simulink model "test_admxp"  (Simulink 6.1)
settings: Solver=ode45  StartTime=0.0  StopTime=2000  RelTol=1e-3
undefined symbols (not defined in the file or in its folder): Bit, Location, Lower, netlist, Width
libraries: xbsIndex_r3 x144, adlibrary2 x7

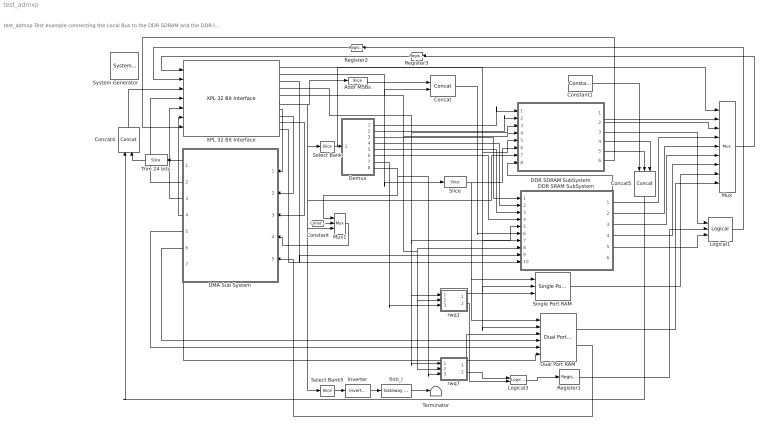
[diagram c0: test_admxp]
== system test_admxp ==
  note: test_admxp Test example connecting the Local Bus to the DDR SDRAM and the DDR-II SSRAM on the ADM-XP
  " System Generator" : xbsIndex_r3/ System Generator  Tag=genX  xilinxfamily=Virtex2P  part=xc2vp70  speed=-5  package=ff1704  synthesis_tool=XST  directory=./netlist  testbench=off  simulink_period=1  sysclk_period=10  incr_netlist=off  trim_vbits=Everywhere in SubSystem  dbl_ovrd=According to Block Masks  core_generation=According to Block Masks  run_coregen=off  deprecated_control=off  eval_field=0
  Addr MSBs : xbsIndex_r3/Slice  mode=Lower Bit Location + Width  nbits=5  bit1=0  base1=MSB of Input  bit0=4  base0=LSB of Input  boolean_output=off  explicit_period=on  period=1  dbl_ovrd=off
  Concat : xbsIndex_r3/Concat  num_inputs=2  explicit_period=on  period=1  dbl_ovrd=off
  Concat4 : xbsIndex_r3/Concat  Orientation=up  num_inputs=2  explicit_period=on  period=1  dbl_ovrd=off
  Concat5 : xbsIndex_r3/Concat  Orientation=down  num_inputs=3  explicit_period=on  period=1  dbl_ovrd=off
  Constant : xbsIndex_r3/Constant  const=0  equ=P=C  arith_type=Unsigned  n_bits=32  bin_pt=0  opselect=C  inp2=PCIN>>17  opr=+  inp1=P  carry=CIN  iostate=0  explicit_period=off  period=1  dbl_ovrd=off
  Constant1 : xbsIndex_r3/Constant  const=0  equ=P=C  arith_type=Unsigned  n_bits=6  bin_pt=0  opselect=C  inp2=PCIN>>17  opr=+  inp1=P  carry=CIN  iostate=0  explicit_period=on  period=1  dbl_ovrd=off
  DDR SDRAM SubSystem : Subsystem
  DDR SRAM SubSystem : Subsystem
  DMA Sub System : Subsystem  Orientation=left
  Demux : Subsystem
  Dual Port RAM : xbsIndex_r3/Dual Port RAM  depth=1024  initVector=sin(pi*(0:15)/16)  write_mode_A=Read After Write  write_mode_B=Read After Write  latency=1  mem_collision=off  init_zero=on  explicit_period=on  period=1  dbl_ovrd=off  rst_a=off  init_a=0  rst_b=off  init_b=0  show_param=off  distributed_mem=off  use_rpm=off  gen_core=off
  Inverter : xbsIndex_r3/Inverter  latency=0  explicit_period=off  period=1  en=off  dbl_ovrd=off  show_param=off
  Logical1 : xbsIndex_r3/Logical  logical_function=OR  inputs=3  precision=Full  arith_type=Unsigned  n_bits=8  bin_pt=2  align_bp=on  latency=0  explicit_period=off  period=1  en=off  dbl_ovrd=off  show_param=off
  Logical3 : xbsIndex_r3/Logical  logical_function=OR  inputs=2  precision=Full  arith_type=Unsigned  n_bits=8  bin_pt=2  align_bp=on  latency=0  explicit_period=off  period=1  en=off  dbl_ovrd=off  show_param=off
  Mux : xbsIndex_r3/Mux  inputs=8  precision=Full  arith_type="Signed  (2's comp)"  n_bits=8  bin_pt=2  quantization=Truncate  overflow=Wrap  latency=0  explicit_period=off  period=1  en=off  dbl_ovrd=off  show_param=off  mux_type=off  use_rpm=off  gen_core=off
  Mux1 : xbsIndex_r3/Mux  inputs=2  precision=Full  arith_type="Signed  (2's comp)"  n_bits=8  bin_pt=2  quantization=Truncate  overflow=Wrap  latency=0  explicit_period=off  period=1  en=off  dbl_ovrd=off  show_param=off  mux_type=off  use_rpm=off  gen_core=off
  Register1 : xbsIndex_r3/Register  init=0  reg_only_valid=off  explicit_period=off  period=1  rst=off  en=off  out_en=off  dbl_ovrd=off  show_param=off
  Register2 : xbsIndex_r3/Register  Orientation=left  init=0  reg_only_valid=off  explicit_period=on  period=1  rst=off  en=off  out_en=off  dbl_ovrd=off  show_param=off
  Register3 : xbsIndex_r3/Register  Orientation=left  init=0  reg_only_valid=off  explicit_period=on  period=1  rst=off  en=off  out_en=off  dbl_ovrd=off  show_param=off
  Select Bank : xbsIndex_r3/Slice  mode=Lower Bit Location + Width  nbits=3  bit1=0  base1=MSB of Input  bit0=0  base0=LSB of Input  boolean_output=off  explicit_period=on  period=1  dbl_ovrd=off
  Select Bank5 : xbsIndex_r3/Slice  mode=Lower Bit Location + Width  nbits=1  bit1=0  base1=MSB of Input  bit0=15  base0=LSB of Input  boolean_output=on  explicit_period=on  period=1  dbl_ovrd=off
  Single Port RAM : xbsIndex_r3/Single Port RAM  depth=1024  initVector=sin(pi*(0:15)/16)  write_mode=Read After Write  latency=1  init_zero=on  explicit_period=off  period=1  rst=off  init_reg=0  en=off  dbl_ovrd=off  show_param=off  distributed_mem=off  use_rpm=off  gen_core=off
  Slice : xbsIndex_r3/Slice  mode=Lower Bit Location + Width  nbits=10  bit1=0  base1=MSB of Input  bit0=0  base0=LSB of Input  boolean_output=off  explicit_period=on  period=1  dbl_ovrd=off
  Terminator : Terminator
  Trim 24 bits : xbsIndex_r3/Slice  Orientation=left  mode=Lower Bit Location + Width  nbits=24  bit1=0  base1=MSB of Input  bit0=0  base0=LSB of Input  boolean_output=off  explicit_period=on  period=1  dbl_ovrd=off
  XPL 32 Bit Interface : adlibrary2/ADM-XP/XPL 32 Bit Interface  program='load test_admxp_program.txt'  clock_ratio=1.5
  finti_l : xbsIndex_r3/Gateway Out  output_type=Double  nbits=8  bin_pt=6  arith_type=Boolean  quantization=Truncate  overflow=Wrap  hdl_port=on  timing_constraint=None  locs_specified=on  LOCs={'AF3'}  needs_fixed_name=off  show_param=off
  rwq1 : Subsystem
  rwq7 : Subsystem
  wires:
  XPL 32 Bit Interface/1 -> DDR SDRAM SubSystem/5(Data), DDR SRAM SubSystem/5(Data), Dual Port RAM/2, Single Port RAM/2
  Register1/1 -> Logical1/2
  Mux/1 -> Register3/1
  Register2/1 -> XPL 32 Bit Interface/2
  Register3/1 -> XPL 32 Bit Interface/1
  Slice/1 -> DDR SDRAM SubSystem/6(Cache Addr), Dual Port RAM/1, Single Port RAM/1
  Addr MSBs/1 -> Concat/1
  XPL 32 Bit Interface/2 -> Concat/2, Slice/1
  Select Bank/1 -> Demux/1(Select), Mux/1
  rwq7/1(wq) -> Dual Port RAM/3
  DMA Sub System/2(Read IFIFO) -> XPL 32 Bit Interface/4
  DMA Sub System/3(Write OFIFO) -> XPL 32 Bit Interface/5
  DMA Sub System/4(OFIFO_Data) -> XPL 32 Bit Interface/6
  Dual Port RAM/2 -> DMA Sub System/5(DP_RAM_Data)
  DMA Sub System/7(DP_RAM_WE) -> Dual Port RAM/6
  DMA Sub System/6(DP_RAM_Addr) -> Dual Port RAM/4
  DMA Sub System/5(DP_RAM_WData) -> Dual Port RAM/5
  Logical1/1 -> Register2/1
  XPL 32 Bit Interface/4 -> DDR SDRAM SubSystem/3(Write), DDR SRAM SubSystem/7(Write), rwq7/1(w), rwq1/1(w)
  XPL 32 Bit Interface/9 -> DMA Sub System/3(OFIFO_Full)
  XPL 32 Bit Interface/8 -> DMA Sub System/2(IFIFO_Empty)
  XPL 32 Bit Interface/7 -> DMA Sub System/1(IFIFO_Data)
  XPL 32 Bit Interface/6 -> Addr MSBs/1, Select Bank/1, DDR SDRAM SubSystem/7(Control), Select Bank5/1, Mux1/3
  XPL 32 Bit Interface/5 -> DDR SRAM SubSystem/8(Read), rwq7/2(r), rwq1/2(r), DDR SDRAM SubSystem/4(Read)
  Concat4/1 -> XPL 32 Bit Interface/3
  DMA Sub System/1(Status) -> Trim 24 bits/1
  Concat5/1 -> Concat4/1
  Select Bank5/1 -> Inverter/1
  finti_l/1 -> Terminator/1
  Concat/1 -> DDR SRAM SubSystem/6(Addr)
  Demux/1(En0) -> DDR SDRAM SubSystem/1(En0)
  Demux/3(En2) -> DDR SRAM SubSystem/1(En2)
  Demux/4(En3) -> DDR SRAM SubSystem/2(En3)
  Demux/5(En4) -> DDR SRAM SubSystem/3(En4)
  Demux/6(En5) -> DDR SRAM SubSystem/4(En5)
  DDR SRAM SubSystem/5(Data Valid) -> Logical1/3
  DDR SDRAM SubSystem/3(Data Valid) -> Logical1/1
  DDR SDRAM SubSystem/1(Data Out0) -> Mux/2
  DDR SDRAM SubSystem/2(Data Out1) -> Mux/3
  Dual Port RAM/1 -> Mux/9
  Demux/7(En6) -> rwq1/3(e)
  Demux/8(En7) -> rwq7/3(e), Mux1/1
  Demux/2(En1) -> DDR SDRAM SubSystem/2(En1)
  Mux1/1 -> DMA Sub System/4(Control)
  Constant/1 -> Mux1/2
  Trim 24 bits/1 -> Concat4/2
  DDR SRAM SubSystem/1(Data Out0) -> Mux/4
  DDR SRAM SubSystem/2(Data Out1) -> Mux/5
  DDR SRAM SubSystem/3(Data Out2) -> Mux/6
  DDR SRAM SubSystem/4(Data Out3) -> Mux/7
  XPL 32 Bit Interface/3 -> DDR SRAM SubSystem/9(be)
  rwq7/2(rq) -> Logical3/1
  Logical3/1 -> Register1/1
  rwq1/2(rq) -> Logical3/2
  rwq1/1(wq) -> Single Port RAM/3
  Single Port RAM/1 -> Mux/8
  XPL 32 Bit Interface/10 -> DDR SRAM SubSystem/10(ADLOCB_IN)
  DDR SRAM SubSystem/6(ADLOCB_OUT) -> DDR SDRAM SubSystem/8(ADLOCB_IN)
  DDR SDRAM SubSystem/6(ADLOCB_OUT) -> XPL 32 Bit Interface/7
  DDR SDRAM SubSystem/4(DDR_Busy0) -> Concat5/3
  DDR SDRAM SubSystem/5(DDR_Busy1) -> Concat5/2
  Constant1/1 -> Concat5/1
  Inverter/1 -> finti_l/1

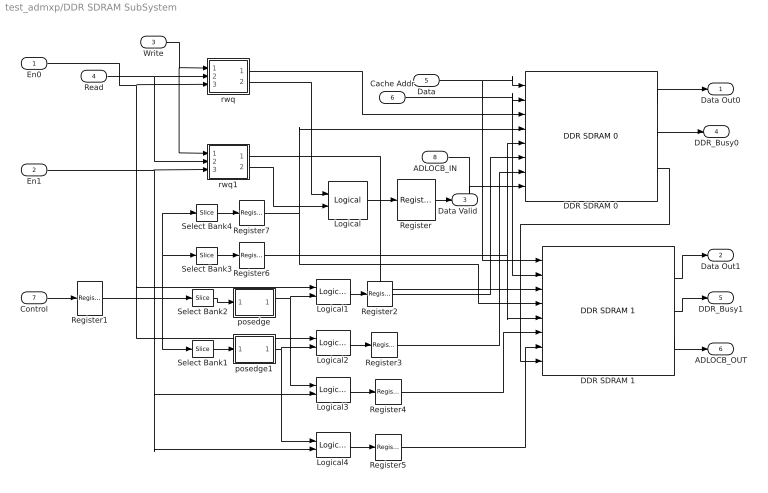
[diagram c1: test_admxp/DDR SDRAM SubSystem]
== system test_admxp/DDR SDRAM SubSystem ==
  En0 : Inport  Port=1  LatchInput=off
  En1 : Inport  Port=2  LatchInput=off
  Write : Inport  Port=3  LatchInput=off
  Read : Inport  Port=4  LatchInput=off
  Data : Inport  Port=5  LatchInput=off
  Cache Addr : Inport  Port=6  LatchInput=off
  Control : Inport  Port=7  LatchInput=off
  ADLOCB_IN : Inport  Port=8  LatchInput=off
  DDR SDRAM 0 : adlibrary2/ADM-XP/DDR SDRAM 0  memsize=1
  DDR SDRAM 1 : adlibrary2/ADM-XP/DDR SDRAM 1  memsize=1
  Logical : xbsIndex_r3/Logical  logical_function=OR  inputs=2  precision=Full  arith_type=Unsigned  n_bits=8  bin_pt=2  align_bp=on  latency=0  explicit_period=off  period=1  en=off  dbl_ovrd=off  show_param=off
  Logical{1..4} (4 alike) : xbsIndex_r3/Logical  logical_function=AND  inputs=2  precision=Full  arith_type=Unsigned  n_bits=8  bin_pt=2  align_bp=on  latency=0  explicit_period=off  period=1  en=off  dbl_ovrd=off  show_param=off
  Register{,2..7} (7 alike) : xbsIndex_r3/Register  init=0  reg_only_valid=off  explicit_period=on  period=1  rst=off  en=off  out_en=off  dbl_ovrd=off  show_param=off
  Register1 : xbsIndex_r3/Register  init=0  reg_only_valid=off  explicit_period=off  period=1  rst=off  en=off  out_en=off  dbl_ovrd=off  show_param=off
  Select Bank1 : xbsIndex_r3/Slice  mode=Lower Bit Location + Width  nbits=1  bit1=0  base1=MSB of Input  bit0=5  base0=LSB of Input  boolean_output=on  explicit_period=on  period=1  dbl_ovrd=off
  Select Bank2 : xbsIndex_r3/Slice  mode=Lower Bit Location + Width  nbits=1  bit1=0  base1=MSB of Input  bit0=4  base0=LSB of Input  boolean_output=on  explicit_period=on  period=1  dbl_ovrd=off
  Select Bank3 : xbsIndex_r3/Slice  mode=Lower Bit Location + Width  nbits=4  bit1=0  base1=MSB of Input  bit0=8  base0=LSB of Input  boolean_output=off  explicit_period=on  period=1  dbl_ovrd=off
  Select Bank4 : xbsIndex_r3/Slice  mode=Lower Bit Location + Width  nbits=15  bit1=0  base1=MSB of Input  bit0=16  base0=LSB of Input  boolean_output=off  explicit_period=on  period=1  dbl_ovrd=off
  posedge : Subsystem
  posedge1 : Subsystem
  rwq : Subsystem
  rwq1 : Subsystem
  Data Out0 : Outport
  Data Out1 : Outport  Port=2
  Data Valid : Outport  Port=3
  DDR_Busy0 : Outport  Port=4
  DDR_Busy1 : Outport  Port=5
  ADLOCB_OUT : Outport  Port=6
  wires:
  DDR SDRAM 0/1 -> Data Out0/1
  DDR SDRAM 0/2 -> DDR_Busy0/1
  En0/1 -> rwq/3(e), Logical1/1, Logical2/1
  En1/1 -> rwq1/3(e), Logical4/2, Logical3/2
  Write/1 -> rwq/1(w), rwq1/1(w)
  Read/1 -> rwq/2(r), rwq1/2(r)
  Data/1 -> DDR SDRAM 0/1, DDR SDRAM 1/1
  Cache Addr/1 -> DDR SDRAM 0/2, DDR SDRAM 1/2
  rwq/1(wq) -> DDR SDRAM 0/3
  rwq1/1(wq) -> DDR SDRAM 1/3
  Logical/1 -> Register/1
  Register/1 -> Data Valid/1
  rwq/2(rq) -> Logical/1
  rwq1/2(rq) -> Logical/2
  Control/1 -> Register1/1
  Select Bank2/1 -> posedge/1(In1)
  Select Bank1/1 -> posedge1/1(In1)
  posedge/1(Out1) -> Logical1/2, Logical3/1
  posedge1/1(Out1) -> Logical2/2, Logical4/1
  Logical1/1 -> Register2/1
  Logical2/1 -> Register3/1
  Logical3/1 -> Register4/1
  Register1/1 -> Select Bank2/1, Select Bank1/1, Select Bank4/1, Select Bank3/1
  Select Bank3/1 -> Register6/1
  Select Bank4/1 -> Register7/1
  Logical4/1 -> Register5/1
  DDR SDRAM 1/1 -> Data Out1/1
  DDR SDRAM 1/2 -> DDR_Busy1/1
  Register2/1 -> DDR SDRAM 0/6
  Register3/1 -> DDR SDRAM 0/7
  Register4/1 -> DDR SDRAM 1/6
  Register5/1 -> DDR SDRAM 1/7
  Register6/1 -> DDR SDRAM 0/5, DDR SDRAM 1/5
  Register7/1 -> DDR SDRAM 0/4, DDR SDRAM 1/4
  ADLOCB_IN/1 -> DDR SDRAM 0/8
  DDR SDRAM 0/3 -> DDR SDRAM 1/8
  DDR SDRAM 1/3 -> ADLOCB_OUT/1

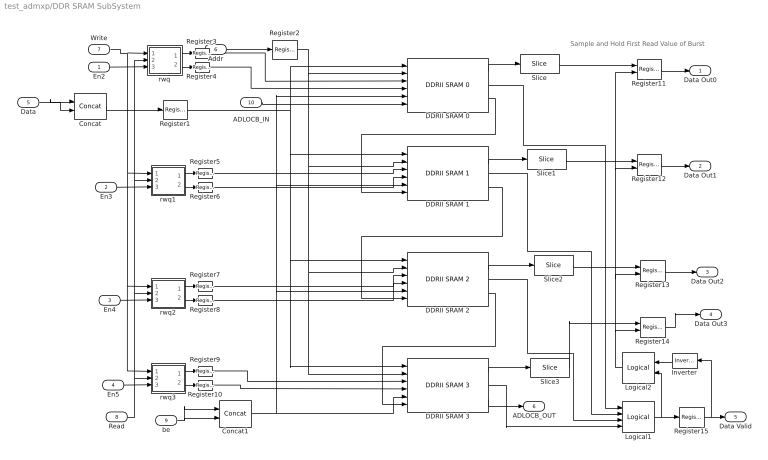
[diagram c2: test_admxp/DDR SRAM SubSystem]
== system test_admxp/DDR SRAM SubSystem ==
  note: Sample and Hold First Read Value of Burst
  En2 : Inport  Port=1  LatchInput=off
  En3 : Inport  Port=2  LatchInput=off
  En4 : Inport  Port=3  LatchInput=off
  En5 : Inport  Port=4  LatchInput=off
  Data : Inport  Port=5  LatchInput=off
  Addr : Inport  Port=6  LatchInput=off
  Write : Inport  Port=7  LatchInput=off
  Read : Inport  Port=8  LatchInput=off
  be : Inport  Port=9  LatchInput=off
  ADLOCB_IN : Inport  Port=10  LatchInput=off
  Concat : xbsIndex_r3/Concat  num_inputs=2  explicit_period=on  period=1  dbl_ovrd=off
  Concat1 : xbsIndex_r3/Concat  num_inputs=2  explicit_period=on  period=1  dbl_ovrd=off
  DDRII SRAM 0 : adlibrary2/ADM-XP/DDRII SRAM 0
  DDRII SRAM 1 : adlibrary2/ADM-XP/DDRII SRAM 1
  DDRII SRAM 2 : adlibrary2/ADM-XP/DDRII SRAM 2
  DDRII SRAM 3 : adlibrary2/ADM-XP/DDRII SRAM 3
  Inverter : xbsIndex_r3/Inverter  Orientation=left  latency=0  explicit_period=off  period=1  en=off  dbl_ovrd=off  show_param=off
  Logical1 : xbsIndex_r3/Logical  logical_function=OR  inputs=4  precision=Full  arith_type=Unsigned  n_bits=8  bin_pt=2  align_bp=on  latency=0  explicit_period=off  period=1  en=off  dbl_ovrd=off  show_param=off
  Logical2 : xbsIndex_r3/Logical  Orientation=left  logical_function=AND  inputs=2  precision=Full  arith_type=Unsigned  n_bits=8  bin_pt=2  align_bp=on  latency=0  explicit_period=off  period=1  en=off  dbl_ovrd=off  show_param=off
  Register{1..10,15} (11 alike) : xbsIndex_r3/Register  init=0  reg_only_valid=off  explicit_period=off  period=1  rst=off  en=off  out_en=off  dbl_ovrd=off  show_param=off
  Register{11..14} (4 alike) : xbsIndex_r3/Register  init=0  reg_only_valid=off  explicit_period=off  period=1  rst=off  en=on  out_en=off  dbl_ovrd=off  show_param=off
  Slice{,1..3} (4 alike) : xbsIndex_r3/Slice  mode=Lower Bit Location + Width  nbits=32  bit1=0  base1=MSB of Input  bit0=0  base0=LSB of Input  boolean_output=off  explicit_period=on  period=1  dbl_ovrd=off
  rwq : Subsystem
  rwq1 : Subsystem
  rwq2 : Subsystem
  rwq3 : Subsystem
  Data Out0 : Outport
  Data Out1 : Outport  Port=2
  Data Out2 : Outport  Port=3
  Data Out3 : Outport  Port=4
  Data Valid : Outport  Port=5
  ADLOCB_OUT : Outport  Port=6
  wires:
  En5/1 -> rwq3/3(e)
  En4/1 -> rwq2/3(e)
  En3/1 -> rwq1/3(e)
  En2/1 -> rwq/3(e)
  Write/1 -> rwq/1(w), rwq3/1(w), rwq2/1(w), rwq1/1(w)
  Read/1 -> rwq3/2(r), rwq/2(r), rwq1/2(r), rwq2/2(r)
  Concat/1 -> Register1/1
  Data/1 -> Concat/1, Concat/2
  Addr/1 -> Register2/1
  rwq/1(wq) -> Register3/1
  rwq/2(rq) -> Register4/1
  rwq1/1(wq) -> Register5/1
  rwq1/2(rq) -> Register6/1
  rwq2/1(wq) -> Register7/1
  rwq2/2(rq) -> Register8/1
  rwq3/1(wq) -> Register9/1
  rwq3/2(rq) -> Register10/1
  be/1 -> Concat1/1, Concat1/2
  DDRII SRAM 0/1 -> Slice/1
  DDRII SRAM 1/1 -> Slice1/1
  DDRII SRAM 2/1 -> Slice2/1
  DDRII SRAM 3/1 -> Slice3/1
  DDRII SRAM 3/2 -> Logical1/4
  Logical1/1 -> Register15/1, Logical2/2
  DDRII SRAM 2/2 -> Logical1/3
  DDRII SRAM 1/2 -> Logical1/2
  DDRII SRAM 0/2 -> Logical1/1
  ADLOCB_IN/1 -> DDRII SRAM 0/6
  DDRII SRAM 0/3 -> DDRII SRAM 1/6
  DDRII SRAM 1/3 -> DDRII SRAM 2/6
  DDRII SRAM 2/3 -> DDRII SRAM 3/6
  DDRII SRAM 3/3 -> ADLOCB_OUT/1
  Concat1/1 -> DDRII SRAM 3/5, DDRII SRAM 2/5, DDRII SRAM 1/5, DDRII SRAM 0/5
  Register1/1 -> DDRII SRAM 0/1, DDRII SRAM 1/1, DDRII SRAM 2/1, DDRII SRAM 3/1
  Register2/1 -> DDRII SRAM 0/2, DDRII SRAM 1/2, DDRII SRAM 2/2, DDRII SRAM 3/2
  Register3/1 -> DDRII SRAM 0/3
  Register4/1 -> DDRII SRAM 0/4
  Register5/1 -> DDRII SRAM 1/3
  Register6/1 -> DDRII SRAM 1/4
  Register7/1 -> DDRII SRAM 2/3
  Register8/1 -> DDRII SRAM 2/4
  Register9/1 -> DDRII SRAM 3/3
  Register10/1 -> DDRII SRAM 3/4
  Slice/1 -> Register11/1
  Register11/1 -> Data Out0/1
  Register12/1 -> Data Out1/1
  Slice1/1 -> Register12/1
  Slice2/1 -> Register13/1
  Register13/1 -> Data Out2/1
  Slice3/1 -> Register14/1
  Register14/1 -> Data Out3/1
  Register15/1 -> Data Valid/1, Inverter/1
  Logical2/1 -> Register14/2, Register13/2, Register12/2, Register11/2
  Inverter/1 -> Logical2/1

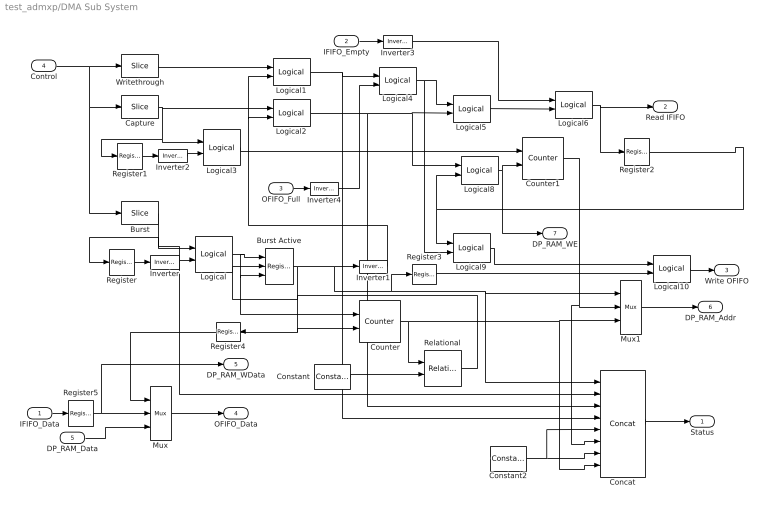
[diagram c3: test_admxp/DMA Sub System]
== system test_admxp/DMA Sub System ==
  IFIFO_Data : Inport  Port=1  LatchInput=off
  IFIFO_Empty : Inport  Port=2  LatchInput=off
  OFIFO_Full : Inport  Port=3  LatchInput=off
  Control : Inport  Port=4  LatchInput=off
  DP_RAM_Data : Inport  Port=5  LatchInput=off
  Burst : xbsIndex_r3/Slice  mode=Lower Bit Location + Width  nbits=1  bit1=0  base1=MSB of Input  bit0=6  base0=LSB of Input  boolean_output=on  explicit_period=on  period=1  dbl_ovrd=off
  Burst Active : xbsIndex_r3/Register  init=0  reg_only_valid=off  explicit_period=on  period=1  rst=on  en=on  out_en=off  dbl_ovrd=off  show_param=off
  Capture : xbsIndex_r3/Slice  mode=Lower Bit Location + Width  nbits=1  bit1=0  base1=MSB of Input  bit0=5  base0=LSB of Input  boolean_output=on  explicit_period=on  period=1  dbl_ovrd=off
  Concat : xbsIndex_r3/Concat  num_inputs=8  explicit_period=on  period=1  dbl_ovrd=off
  Constant : xbsIndex_r3/Constant  const=511  equ=P=C  arith_type=Unsigned  n_bits=10  bin_pt=0  opselect=C  inp2=PCIN>>17  opr=+  inp1=P  carry=CIN  iostate=0  explicit_period=off  period=1  dbl_ovrd=off
  Constant2 : xbsIndex_r3/Constant  const=0  equ=P=C  arith_type=Unsigned  n_bits=2  bin_pt=0  opselect=C  inp2=PCIN>>17  opr=+  inp1=P  carry=CIN  iostate=0  explicit_period=off  period=1  dbl_ovrd=off
  Counter : xbsIndex_r3/Counter  cnt_type=Count Limited  n_bits=10  bin_pt=0  arith_type=Unsigned  start_count=0  cnt_to=Inf  cnt_by_val=1  operation=Up  explicit_period=on  period=1  load_pin=off  rst=on  en=on  dbl_ovrd=off  show_param=off  use_rpm=on  gen_core=off
  Counter1 : xbsIndex_r3/Counter  cnt_type=Count Limited  n_bits=10  bin_pt=0  arith_type=Unsigned  start_count=0  cnt_to=Inf  cnt_by_val=1  operation=Up  explicit_period=on  period=1  load_pin=off  rst=on  en=on  dbl_ovrd=off  show_param=off  use_rpm=on  gen_core=off
  Inverter{,1..2,4} (4 alike) : xbsIndex_r3/Inverter  latency=0  explicit_period=off  period=1  en=off  dbl_ovrd=off  show_param=off
  Inverter3 : xbsIndex_r3/Inverter  latency=0  explicit_period=on  period=1  en=off  dbl_ovrd=off  show_param=off
  Logical : xbsIndex_r3/Logical  logical_function=AND  inputs=2  precision=Full  arith_type=Unsigned  n_bits=8  bin_pt=2  align_bp=on  latency=0  explicit_period=on  period=1  en=off  dbl_ovrd=off  show_param=off
  Logical{1..2,4,8..9} (5 alike) : xbsIndex_r3/Logical  logical_function=AND  inputs=2  precision=Full  arith_type=Unsigned  n_bits=8  bin_pt=2  align_bp=on  latency=0  explicit_period=off  period=1  en=off  dbl_ovrd=off  show_param=off
  Logical10 : xbsIndex_r3/Logical  logical_function=OR  inputs=2  precision=Full  arith_type=Unsigned  n_bits=8  bin_pt=2  align_bp=on  latency=0  explicit_period=on  period=1  en=off  dbl_ovrd=off  show_param=off
  Logical3 : xbsIndex_r3/Logical  logical_function=AND  inputs=2  precision=Full  arith_type=Unsigned  n_bits=8  bin_pt=2  align_bp=on  latency=0  explicit_period=on  period=1  en=off  dbl_ovrd=off  show_param=off
  Logical5 : xbsIndex_r3/Logical  logical_function=OR  inputs=2  precision=Full  arith_type=Unsigned  n_bits=8  bin_pt=2  align_bp=on  latency=0  explicit_period=off  period=1  en=off  dbl_ovrd=off  show_param=off
  Logical6 : xbsIndex_r3/Logical  logical_function=AND  inputs=2  precision=Full  arith_type=Unsigned  n_bits=8  bin_pt=2  align_bp=on  latency=0  explicit_period=on  period=1  en=off  dbl_ovrd=off  show_param=off
  Mux : xbsIndex_r3/Mux  inputs=2  precision=Full  arith_type="Signed  (2's comp)"  n_bits=8  bin_pt=2  quantization=Truncate  overflow=Wrap  latency=0  explicit_period=on  period=1  en=off  dbl_ovrd=off  show_param=off  mux_type=off  use_rpm=off  gen_core=off
  Mux1 : xbsIndex_r3/Mux  inputs=2  precision=Full  arith_type="Signed  (2's comp)"  n_bits=8  bin_pt=2  quantization=Truncate  overflow=Wrap  latency=0  explicit_period=off  period=1  en=off  dbl_ovrd=off  show_param=off  mux_type=off  use_rpm=off  gen_core=off
  Register{,1..3,5} (5 alike) : xbsIndex_r3/Register  init=0  reg_only_valid=off  explicit_period=on  period=1  rst=off  en=off  out_en=off  dbl_ovrd=off  show_param=off
  Register4 : xbsIndex_r3/Register  Orientation=left  init=0  reg_only_valid=off  explicit_period=on  period=1  rst=off  en=off  out_en=off  dbl_ovrd=off  show_param=off
  Relational : xbsIndex_r3/Relational  mode=a=b  latency=0  explicit_period=off  period=1  en=off  dbl_ovrd=off  show_param=off
  Writethrough : xbsIndex_r3/Slice  mode=Lower Bit Location + Width  nbits=1  bit1=0  base1=MSB of Input  bit0=4  base0=LSB of Input  boolean_output=on  explicit_period=on  period=1  dbl_ovrd=off
  Status : Outport
  Read IFIFO : Outport  Port=2
  Write OFIFO : Outport  Port=3
  OFIFO_Data : Outport  Port=4
  DP_RAM_WData : Outport  Port=5
  DP_RAM_Addr : Outport  Port=6
  DP_RAM_WE : Outport  Port=7
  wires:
  Mux/1 -> OFIFO_Data/1
  IFIFO_Data/1 -> Register5/1
  DP_RAM_Data/1 -> Mux/3
  Control/1 -> Writethrough/1, Burst/1, Capture/1
  Burst/1 -> Register/1, Logical/1, Concat/2
  Register/1 -> Inverter/1
  Inverter/1 -> Logical/2
  Logical/1 -> Burst Active/1, Burst Active/3, Counter/1
  Burst Active/1 -> Inverter1/1, Register3/1, Mux1/1, Concat/1, Counter/2, Register4/1
  Inverter1/1 -> Logical1/2, Logical2/2
  Capture/1 -> Logical2/1, Logical3/1, Register1/1
  Writethrough/1 -> Logical1/1
  Register1/1 -> Inverter2/1
  Inverter2/1 -> Logical3/2
  Logical3/1 -> Counter1/1
  IFIFO_Empty/1 -> Inverter3/1
  OFIFO_Full/1 -> Inverter4/1
  Logical1/1 -> Logical4/1, Concat/4
  Inverter4/1 -> Logical4/2
  Logical2/1 -> Logical5/2, Logical8/1, Concat/3
  Logical4/1 -> Logical5/1, Logical9/2
  Inverter3/1 -> Logical6/1
  Logical5/1 -> Logical6/2
  Logical6/1 -> Read IFIFO/1, Register2/1
  Register2/1 -> Logical8/2, Logical9/1
  Logical8/1 -> Counter1/2, DP_RAM_WE/1
  Mux1/1 -> DP_RAM_Addr/1
  Counter1/1 -> Mux1/2, Concat/6
  Counter/1 -> Relational/1, Mux1/3, Concat/8
  Logical9/1 -> Logical10/1
  Register3/1 -> Logical10/2
  Constant/1 -> Relational/2
  Relational/1 -> Burst Active/2
  Constant2/1 -> Concat/5, Concat/7
  Concat/1 -> Status/1
  Logical10/1 -> Write OFIFO/1
  Register4/1 -> Mux/1
  Register5/1 -> Mux/2, DP_RAM_WData/1

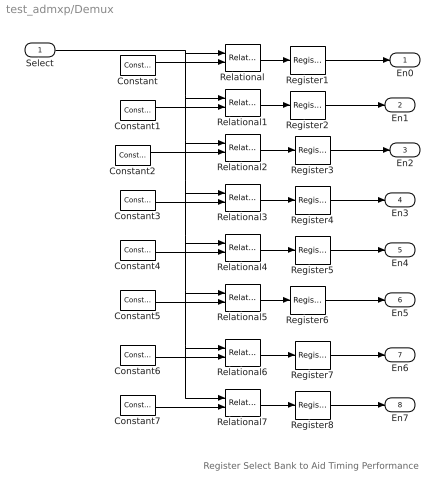
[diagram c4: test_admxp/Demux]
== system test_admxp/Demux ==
  note: Register Select Bank to Aid Timing Performance
  Select : Inport  Port=1  LatchInput=off
  Constant : xbsIndex_r3/Constant  const=0  equ=P=C  arith_type=Unsigned  n_bits=3  bin_pt=0  opselect=C  inp2=PCIN>>17  opr=+  inp1=P  carry=CIN  iostate=0  explicit_period=off  period=1  dbl_ovrd=off
  Constant1 : xbsIndex_r3/Constant  const=1  equ=P=C  arith_type=Unsigned  n_bits=3  bin_pt=0  opselect=C  inp2=PCIN>>17  opr=+  inp1=P  carry=CIN  iostate=0  explicit_period=off  period=1  dbl_ovrd=off
  Constant2 : xbsIndex_r3/Constant  const=2  equ=P=C  arith_type=Unsigned  n_bits=3  bin_pt=0  opselect=C  inp2=PCIN>>17  opr=+  inp1=P  carry=CIN  iostate=0  explicit_period=off  period=1  dbl_ovrd=off
  Constant3 : xbsIndex_r3/Constant  const=3  equ=P=C  arith_type=Unsigned  n_bits=3  bin_pt=0  opselect=C  inp2=PCIN>>17  opr=+  inp1=P  carry=CIN  iostate=0  explicit_period=off  period=1  dbl_ovrd=off
  Constant4 : xbsIndex_r3/Constant  const=4  equ=P=C  arith_type=Unsigned  n_bits=3  bin_pt=0  opselect=C  inp2=PCIN>>17  opr=+  inp1=P  carry=CIN  iostate=0  explicit_period=off  period=1  dbl_ovrd=off
  Constant5 : xbsIndex_r3/Constant  const=5  equ=P=C  arith_type=Unsigned  n_bits=3  bin_pt=0  opselect=C  inp2=PCIN>>17  opr=+  inp1=P  carry=CIN  iostate=0  explicit_period=off  period=1  dbl_ovrd=off
  Constant6 : xbsIndex_r3/Constant  const=6  equ=P=C  arith_type=Unsigned  n_bits=3  bin_pt=0  opselect=C  inp2=PCIN>>17  opr=+  inp1=P  carry=CIN  iostate=0  explicit_period=off  period=1  dbl_ovrd=off
  Constant7 : xbsIndex_r3/Constant  const=7  equ=P=C  arith_type=Unsigned  n_bits=3  bin_pt=0  opselect=C  inp2=PCIN>>17  opr=+  inp1=P  carry=CIN  iostate=0  explicit_period=off  period=1  dbl_ovrd=off
  Register{1..8} (8 alike) : xbsIndex_r3/Register  init=0  reg_only_valid=off  explicit_period=off  period=1  rst=off  en=off  out_en=off  dbl_ovrd=off  show_param=off
  Relational{,1..7} (8 alike) : xbsIndex_r3/Relational  mode=a=b  latency=0  explicit_period=off  period=1  en=off  dbl_ovrd=off  show_param=off
  En0 : Outport
  En1 : Outport  Port=2
  En2 : Outport  Port=3
  En3 : Outport  Port=4
  En4 : Outport  Port=5
  En5 : Outport  Port=6
  En6 : Outport  Port=7
  En7 : Outport  Port=8
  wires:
  Relational/1 -> Register1/1
  Relational1/1 -> Register2/1
  Relational2/1 -> Register3/1
  Relational3/1 -> Register4/1
  Select/1 -> Relational/1, Relational1/1, Relational2/1, Relational3/1, Relational4/1, Relational5/1, Relational6/1, Relational7/1
  Constant/1 -> Relational/2
  Constant1/1 -> Relational1/2
  Constant2/1 -> Relational2/2
  Constant3/1 -> Relational3/2
  Relational4/1 -> Register5/1
  Constant4/1 -> Relational4/2
  Relational5/1 -> Register6/1
  Constant5/1 -> Relational5/2
  Relational6/1 -> Register7/1
  Constant6/1 -> Relational6/2
  Relational7/1 -> Register8/1
  Constant7/1 -> Relational7/2
  Register1/1 -> En0/1
  Register2/1 -> En1/1
  Register3/1 -> En2/1
  Register4/1 -> En3/1
  Register5/1 -> En4/1
  Register6/1 -> En5/1
  Register7/1 -> En6/1
  Register8/1 -> En7/1

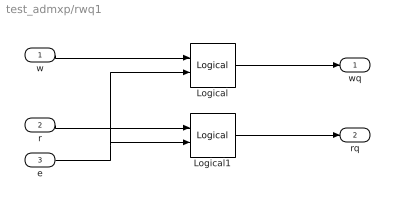
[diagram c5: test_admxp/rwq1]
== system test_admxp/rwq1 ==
  w : Inport  Port=1  LatchInput=off
  r : Inport  Port=2  LatchInput=off
  e : Inport  Port=3  LatchInput=off
  Logical : xbsIndex_r3/Logical  logical_function=AND  inputs=2  precision=Full  arith_type=Unsigned  n_bits=8  bin_pt=2  align_bp=on  latency=0  explicit_period=off  period=1  en=off  dbl_ovrd=off  show_param=off
  Logical1 : xbsIndex_r3/Logical  logical_function=AND  inputs=2  precision=Full  arith_type=Unsigned  n_bits=8  bin_pt=2  align_bp=on  latency=0  explicit_period=off  period=1  en=off  dbl_ovrd=off  show_param=off
  wq : Outport
  rq : Outport  Port=2
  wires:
  e/1 -> Logical1/2, Logical/2
  r/1 -> Logical1/1
  w/1 -> Logical/1
  Logical/1 -> wq/1
  Logical1/1 -> rq/1

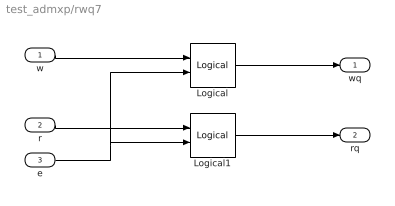
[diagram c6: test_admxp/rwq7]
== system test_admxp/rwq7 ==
  w : Inport  Port=1  LatchInput=off
  r : Inport  Port=2  LatchInput=off
  e : Inport  Port=3  LatchInput=off
  Logical : xbsIndex_r3/Logical  logical_function=AND  inputs=2  precision=Full  arith_type=Unsigned  n_bits=8  bin_pt=2  align_bp=on  latency=0  explicit_period=off  period=1  en=off  dbl_ovrd=off  show_param=off
  Logical1 : xbsIndex_r3/Logical  logical_function=AND  inputs=2  precision=Full  arith_type=Unsigned  n_bits=8  bin_pt=2  align_bp=on  latency=0  explicit_period=off  period=1  en=off  dbl_ovrd=off  show_param=off
  wq : Outport
  rq : Outport  Port=2
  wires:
  e/1 -> Logical1/2, Logical/2
  r/1 -> Logical1/1
  w/1 -> Logical/1
  Logical/1 -> wq/1
  Logical1/1 -> rq/1

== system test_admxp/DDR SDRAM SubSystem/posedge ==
  In1 : Inport  Port=1  LatchInput=off
  Inverter : xbsIndex_r3/Inverter  latency=0  explicit_period=off  period=1  en=off  dbl_ovrd=off  show_param=off
  Logical : xbsIndex_r3/Logical  logical_function=AND  inputs=2  precision=Full  arith_type=Unsigned  n_bits=8  bin_pt=2  align_bp=on  latency=0  explicit_period=off  period=1  en=off  dbl_ovrd=off  show_param=off
  Register : xbsIndex_r3/Register  init=0  reg_only_valid=off  explicit_period=on  period=1  rst=off  en=off  out_en=off  dbl_ovrd=off  show_param=off
  Register1 : xbsIndex_r3/Register  init=0  reg_only_valid=off  explicit_period=on  period=1  rst=off  en=off  out_en=off  dbl_ovrd=off  show_param=off
  Out1 : Outport
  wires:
  Inverter/1 -> Logical/1
  Logical/1 -> Out1/1
  Register/1 -> Logical/2
  In1/1 -> Register1/1
  Register1/1 -> Inverter/1, Register/1

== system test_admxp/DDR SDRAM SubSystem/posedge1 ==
  In1 : Inport  Port=1  LatchInput=off
  Inverter : xbsIndex_r3/Inverter  latency=0  explicit_period=off  period=1  en=off  dbl_ovrd=off  show_param=off
  Logical : xbsIndex_r3/Logical  logical_function=AND  inputs=2  precision=Full  arith_type=Unsigned  n_bits=8  bin_pt=2  align_bp=on  latency=0  explicit_period=off  period=1  en=off  dbl_ovrd=off  show_param=off
  Register : xbsIndex_r3/Register  init=0  reg_only_valid=off  explicit_period=on  period=1  rst=off  en=off  out_en=off  dbl_ovrd=off  show_param=off
  Register1 : xbsIndex_r3/Register  init=0  reg_only_valid=off  explicit_period=on  period=1  rst=off  en=off  out_en=off  dbl_ovrd=off  show_param=off
  Out1 : Outport
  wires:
  Inverter/1 -> Logical/1
  Logical/1 -> Out1/1
  Register/1 -> Logical/2
  In1/1 -> Register1/1
  Register1/1 -> Inverter/1, Register/1

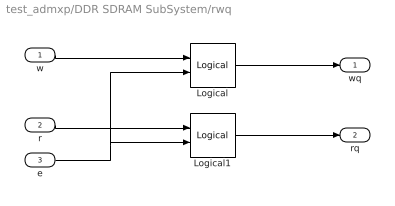
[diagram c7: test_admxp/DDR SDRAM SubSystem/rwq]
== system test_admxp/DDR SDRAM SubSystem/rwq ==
  w : Inport  Port=1  LatchInput=off
  r : Inport  Port=2  LatchInput=off
  e : Inport  Port=3  LatchInput=off
  Logical : xbsIndex_r3/Logical  logical_function=AND  inputs=2  precision=Full  arith_type=Unsigned  n_bits=8  bin_pt=2  align_bp=on  latency=0  explicit_period=off  period=1  en=off  dbl_ovrd=off  show_param=off
  Logical1 : xbsIndex_r3/Logical  logical_function=AND  inputs=2  precision=Full  arith_type=Unsigned  n_bits=8  bin_pt=2  align_bp=on  latency=0  explicit_period=off  period=1  en=off  dbl_ovrd=off  show_param=off
  wq : Outport
  rq : Outport  Port=2
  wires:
  e/1 -> Logical1/2, Logical/2
  r/1 -> Logical1/1
  w/1 -> Logical/1
  Logical/1 -> wq/1
  Logical1/1 -> rq/1

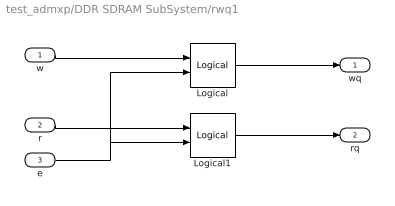
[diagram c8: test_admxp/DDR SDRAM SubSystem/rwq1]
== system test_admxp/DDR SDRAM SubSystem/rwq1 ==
  w : Inport  Port=1  LatchInput=off
  r : Inport  Port=2  LatchInput=off
  e : Inport  Port=3  LatchInput=off
  Logical : xbsIndex_r3/Logical  logical_function=AND  inputs=2  precision=Full  arith_type=Unsigned  n_bits=8  bin_pt=2  align_bp=on  latency=0  explicit_period=off  period=1  en=off  dbl_ovrd=off  show_param=off
  Logical1 : xbsIndex_r3/Logical  logical_function=AND  inputs=2  precision=Full  arith_type=Unsigned  n_bits=8  bin_pt=2  align_bp=on  latency=0  explicit_period=off  period=1  en=off  dbl_ovrd=off  show_param=off
  wq : Outport
  rq : Outport  Port=2
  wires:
  e/1 -> Logical1/2, Logical/2
  r/1 -> Logical1/1
  w/1 -> Logical/1
  Logical/1 -> wq/1
  Logical1/1 -> rq/1

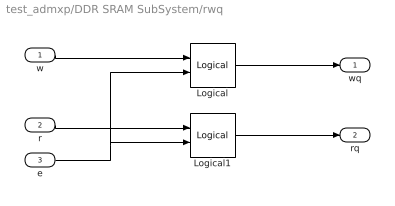
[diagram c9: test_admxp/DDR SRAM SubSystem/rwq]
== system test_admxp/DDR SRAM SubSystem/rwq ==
  w : Inport  Port=1  LatchInput=off
  r : Inport  Port=2  LatchInput=off
  e : Inport  Port=3  LatchInput=off
  Logical : xbsIndex_r3/Logical  logical_function=AND  inputs=2  precision=Full  arith_type=Unsigned  n_bits=8  bin_pt=2  align_bp=on  latency=0  explicit_period=off  period=1  en=off  dbl_ovrd=off  show_param=off
  Logical1 : xbsIndex_r3/Logical  logical_function=AND  inputs=2  precision=Full  arith_type=Unsigned  n_bits=8  bin_pt=2  align_bp=on  latency=0  explicit_period=off  period=1  en=off  dbl_ovrd=off  show_param=off
  wq : Outport
  rq : Outport  Port=2
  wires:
  e/1 -> Logical1/2, Logical/2
  r/1 -> Logical1/1
  w/1 -> Logical/1
  Logical/1 -> wq/1
  Logical1/1 -> rq/1

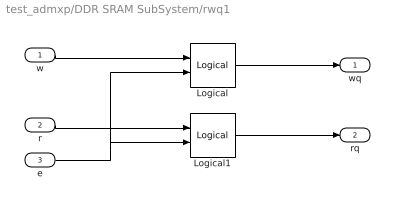
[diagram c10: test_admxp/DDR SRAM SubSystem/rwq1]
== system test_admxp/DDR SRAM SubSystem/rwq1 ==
  w : Inport  Port=1  LatchInput=off
  r : Inport  Port=2  LatchInput=off
  e : Inport  Port=3  LatchInput=off
  Logical : xbsIndex_r3/Logical  logical_function=AND  inputs=2  precision=Full  arith_type=Unsigned  n_bits=8  bin_pt=2  align_bp=on  latency=0  explicit_period=off  period=1  en=off  dbl_ovrd=off  show_param=off
  Logical1 : xbsIndex_r3/Logical  logical_function=AND  inputs=2  precision=Full  arith_type=Unsigned  n_bits=8  bin_pt=2  align_bp=on  latency=0  explicit_period=off  period=1  en=off  dbl_ovrd=off  show_param=off
  wq : Outport
  rq : Outport  Port=2
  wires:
  e/1 -> Logical1/2, Logical/2
  r/1 -> Logical1/1
  w/1 -> Logical/1
  Logical/1 -> wq/1
  Logical1/1 -> rq/1

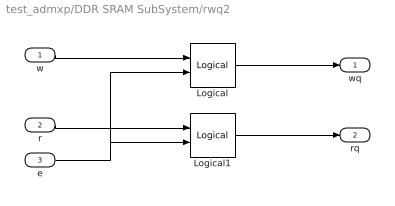
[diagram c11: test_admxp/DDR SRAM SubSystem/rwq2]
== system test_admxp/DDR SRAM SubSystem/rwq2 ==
  w : Inport  Port=1  LatchInput=off
  r : Inport  Port=2  LatchInput=off
  e : Inport  Port=3  LatchInput=off
  Logical : xbsIndex_r3/Logical  logical_function=AND  inputs=2  precision=Full  arith_type=Unsigned  n_bits=8  bin_pt=2  align_bp=on  latency=0  explicit_period=off  period=1  en=off  dbl_ovrd=off  show_param=off
  Logical1 : xbsIndex_r3/Logical  logical_function=AND  inputs=2  precision=Full  arith_type=Unsigned  n_bits=8  bin_pt=2  align_bp=on  latency=0  explicit_period=off  period=1  en=off  dbl_ovrd=off  show_param=off
  wq : Outport
  rq : Outport  Port=2
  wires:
  e/1 -> Logical1/2, Logical/2
  r/1 -> Logical1/1
  w/1 -> Logical/1
  Logical/1 -> wq/1
  Logical1/1 -> rq/1

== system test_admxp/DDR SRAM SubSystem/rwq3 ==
  w : Inport  Port=1  LatchInput=off
  r : Inport  Port=2  LatchInput=off
  e : Inport  Port=3  LatchInput=off
  Logical : xbsIndex_r3/Logical  logical_function=AND  inputs=2  precision=Full  arith_type=Unsigned  n_bits=8  bin_pt=2  align_bp=on  latency=0  explicit_period=off  period=1  en=off  dbl_ovrd=off  show_param=off
  Logical1 : xbsIndex_r3/Logical  logical_function=AND  inputs=2  precision=Full  arith_type=Unsigned  n_bits=8  bin_pt=2  align_bp=on  latency=0  explicit_period=off  period=1  en=off  dbl_ovrd=off  show_param=off
  wq : Outport
  rq : Outport  Port=2
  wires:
  e/1 -> Logical1/2, Logical/2
  r/1 -> Logical1/1
  w/1 -> Logical/1
  Logical/1 -> wq/1
  Logical1/1 -> rq/1
